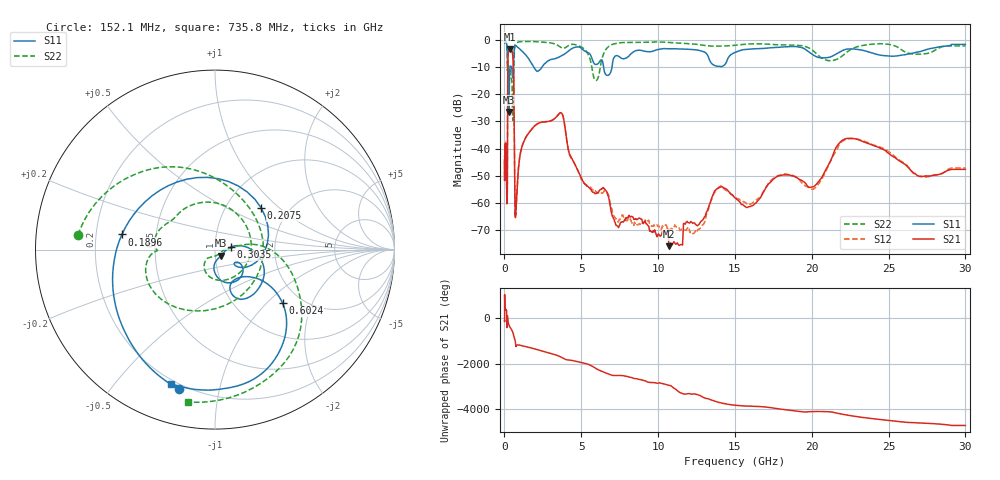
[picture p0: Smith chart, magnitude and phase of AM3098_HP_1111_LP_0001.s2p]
! Date/Time: Thu, Feb 28, 2019 8:47 AM
! Network Analyzer: Agilent Technologies E8364B Rev: A.07.50.67
! Sweep from 0.010 to 30.000 GHz, 1601 Points, Sweep Type: LOG
! Power Supply: 5.022 V, 0.002 A
# Hz S DB R 50
!freq MagS11 AngS11 MagS21 AngS21 MagS12 AngS12 MagS22 AngS22
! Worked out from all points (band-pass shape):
!   1601 points, 10 MHz to 30 GHz, reference 50 ohm
!   highest |S21| = -3.33 dB at 333.7 MHz (marker M1); lowest = -75.9 dB at 10.7 GHz (marker M2)
!   |S21| within 3 dB of the highest: 228.1 MHz to 551.7 MHz (323.5 MHz wide, 83 % of centre)
!   lowest |S11| = -26.5 dB at 288.7 MHz (marker M3), VSWR 1.10, Z = 53.3 - j3.6 ohm
!   |S11| at or under -10 dB: 210 MHz to 373.7 MHz (163.7 MHz wide, 56.1 % of centre); 1.898 GHz to 2.44 GHz (542 MHz wide, 25 % of centre); 6.453 GHz to 7 GHz (547.3 MHz wide, 8.14 % of centre)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
!   |S22| runs from -29.6 to -0.5 dB; largest |S21 - S12| = 0.013
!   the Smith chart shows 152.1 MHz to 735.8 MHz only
!   S11 on the Smith chart (normalised r, x): 152.1 MHz: 0.18, -0.76; 189.6 MHz: 0.31, +0.07; 207.5 MHz: 1.45, +0.77; 303.5 MHz: 1.19, +0.03; 602.4 MHz: 1.61, -1.25; 735.8 MHz: 0.18, -0.71
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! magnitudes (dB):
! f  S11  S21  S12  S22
! 10 MHz  -0.3  -44.9  -42.9  -0.5
! 38.04 MHz  -0.2  -41.6  -40.8  -0.5
! 94.57 MHz  -0.8  -38.9  -39.2  -1.1
! 144.7 MHz  -1.6  -56.1  -54.9  -2.0
! 152.1 MHz  -1.9  -60.1  -57.1  -2.3
! 189.6 MHz  -5.6  -52.3  -52.1  -9.6
! 207.5 MHz  -9.2  -20.3  -20.2  -8.5
! 288.7 MHz  -26.5  -3.5  -3.5  -10.4
! 303.5 MHz  -21.1  -3.4  -3.4  -10.8
! 333.7 MHz  -12.3  -3.3  -3.3  -10.9
! 550.5 MHz  -13.3  -6.3  -6.2  -29.4
! 602.4 MHz  -6.4  -14.4  -14.4  -12.4
! 679.2 MHz  -2.2  -58.5  -60.3  -2.2
! 735.8 MHz  -2.1  -64.0  -64.1  -1.3
! 1.039 GHz  -3.6  -41.7  -41.5  -0.7
! 2.084 GHz  -11.5  -31.1  -31.1  -0.7
! 3.704 GHz  -5.9  -26.9  -26.9  -2.9
! 5.959 GHz  -9.1  -56.5  -55.9  -15.0
! 7.926 GHz  -6.7  -65.6  -66.5  -1.0
! 10.7 GHz  -3.3  -75.9  -69.9  -0.9
! 22.44 GHz  -3.3  -36.2  -36.3  -3.9
! 30 GHz  -1.7  -47.6  -47.1  -2.2
